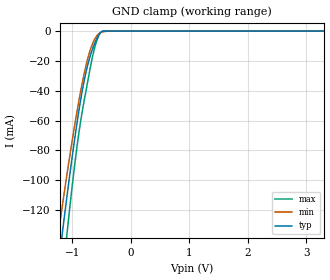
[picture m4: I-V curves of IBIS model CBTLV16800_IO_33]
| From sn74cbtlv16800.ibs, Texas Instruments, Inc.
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[Model]   CBTLV16800_IO_33
Model_type  Terminator
| variable   typ   min   max
C_comp   4.32pF   3.75pF   4.86pF
| C_tri-state   4.32pF   3.75pF   4.86pF
[Temperature Range]   40   100   -40
| Ambient temperature   25   85   -40
[Voltage range]   3.3   3   3.6
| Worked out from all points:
|   GND clamp passes 1 mA (typ) near -0.52 V on its own axis
[GND Clamp]
| CBTLV16800_IO_33
|   Voltage   I(typ)   I(min)   I(max)
-3.3V     -903.9mA   -778.3mA   -1.091A
-1.255V   -163.3mA   -141.1mA   -199.6mA
-1.225V   -153.6mA   -132.7mA   -187.9mA
-1.165V   -134.5mA   -116.3mA   -164.6mA
-1.085V   -109.6mA   -95.11mA   -134.6mA
-910mV    -59.82mA   -52.25mA   -75.36mA
-770mV    -28.68mA   -24.22mA   -41.38mA
-690mV    -16.57mA   -12.61mA   -24.54mA
-615mV    -8.238mA   -5.459mA   -11.11mA
-545mV    -2.536mA   -1.76mA    -3.08mA
-485mV    -154uA     -600.6uA   -132.5uA
3.3V      1.257nA    61.35nA    15.91pA
